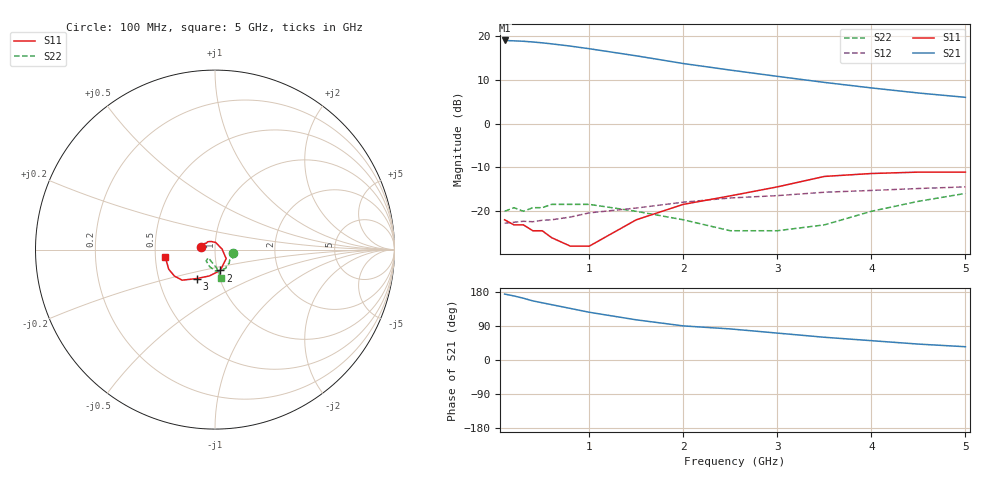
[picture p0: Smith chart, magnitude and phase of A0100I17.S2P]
!  MSA-0100 S AND NOISE PARAMETERS
!  Id = 17 mA  LAST UPDATED 07-22-92
# ghz s ma r 50
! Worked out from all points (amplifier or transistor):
!   16 points, 100 MHz to 5 GHz, reference 50 ohm
!   highest |S21| = 19.0 dB at 100 MHz (marker M1)
!   |S21| within 3 dB of that: start of sweep to 1.343 GHz
!   unconditionally stable (mu >= 1): start of sweep to end of sweep
!   at 300 MHz: K = 1.07, MAG = 19.0 dB, |S12| = -22.3 dB
!   at 1.5 GHz: K = 1.08, MAG = 15.6 dB, |S12| = -19.3 dB
!   at 5 GHz: K = 1.34, MAG = 6.7 dB, |S12| = -14.4 dB
!   lowest NFmin = 5.20 dB at 100 MHz
!   S11 on the Smith chart (normalised r, x): 100 MHz: 0.85, +0.02; 2 GHz: 1.03, -0.24; 3 GHz: 0.78, -0.26; 5 GHz: 0.56, -0.05
0.1  0.08 171.0  8.91 174.0  0.073 2.0  0.1 -11.0
0.2  0.07 161.0  8.82 169.0  0.075 6.0  0.11 -24.0
0.3  0.07 152.0  8.72 163.0  0.077 9.0  0.1 -35.0
0.4  0.06 143.0  8.56 156.0  0.076 12.0  0.11 -44.0
0.5  0.06 133.0  8.37 151.0  0.079 14.0  0.11 -53.0
0.6  0.05 115.0  8.15 146.0  0.08 19.0  0.12 -60.0
0.8  0.04 84.0  7.68 136.0  0.086 22.0  0.12 -75.0
1  0.04 3.0  7.17 126.0  0.096 26.0  0.12 -88.0
1.5  0.08 -39.0  5.95 106.0  0.109 32.0  0.1 -107.0
2  0.12 -76.0  4.86 90.0  0.127 32.0  0.08 -128.0
2.5  0.15 -102.0  4.09 82.0  0.142 36.0  0.06 -130.0
3  0.19 -122.0  3.47 71.0  0.151 36.0  0.06 -125.0
3.5  0.25 -137.0  2.96 60.0  0.165 34.0  0.07 -107.0
4  0.27 -147.0  2.56 51.0  0.173 32.0  0.1 -86.0
4.5  0.28 -157.0  2.24 42.0  0.182 29.0  0.13 -80.0
5  0.28 -171.0  2 35.0  0.19 28.0  0.16 -77.0
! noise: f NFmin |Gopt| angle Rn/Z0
0.1  5.2  0.23  1  1.11
0.5  5.3  0.23  4  1.11
1  5.4  0.21  8  1.1
2  5.8  0.18  16  1.06
